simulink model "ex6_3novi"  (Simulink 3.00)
settings: Solver=VariableStepDiscrete  SolverMode=SingleTasking  StartTime=0.0  StopTime=20  RelTol=1e-3  AbsTol=1e-6

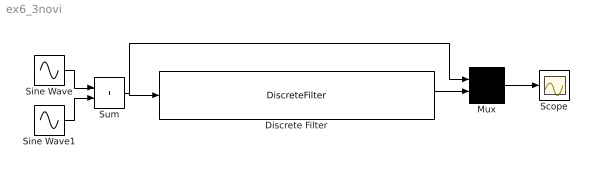
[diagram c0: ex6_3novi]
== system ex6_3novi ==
  Discrete Filter : DiscreteFilter  Numerator="[0.0048 0.0193  0.0289  0.0193  0.0048]"  Denominator="[1.0000  -2.3695  2.3140 -1.0547  0.1874]"  SampleTime=.1
  Mux : Mux  Inputs=2
  Scope : Scope
  Sine Wave : Sin  Amplitude=1  Frequency=0.5  Phase=0  SampleTime=0
  Sine Wave1 : Sin  Amplitude=0.4  Frequency=10  Phase=0  SampleTime=0
  Sum : Sum  Inputs=++  SaturateOnIntegerOverflow=on
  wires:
  Sum/1 -> Discrete Filter/1, Mux/1
  Discrete Filter/1 -> Mux/2
  Sine Wave1/1 -> Sum/2
  Sine Wave/1 -> Sum/1
  Mux/1 -> Scope/1
